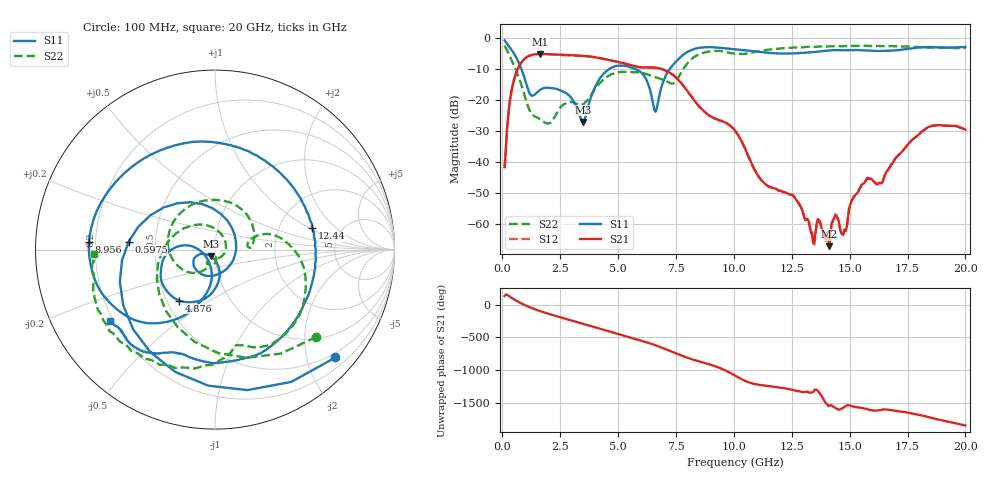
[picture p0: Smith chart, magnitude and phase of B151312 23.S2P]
!  2-Port S-parameters saved by WinCal
! VAR MeasName=S-Parameters (CALIBRATED_DATA) read from VNA (N5244A)
! VAR MeasDate=12/8/2015 5:45:11 PM
! VAR NAME=B151312 23
! VAR FILENAME=B151312 23.S2P
! VAR DATE=12/8/2015 5:45:11 PM
! VAR PHYS_PORTS=1,2
# Hz S DB R 50
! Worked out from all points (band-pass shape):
!   401 points, 100 MHz to 20 GHz, reference 50 ohm
!   highest |S21| = -5.26 dB at 1.642 GHz (marker M1); lowest = -67.2 dB at 14.13 GHz (marker M2)
!   |S21| within 3 dB of the highest: 802.2 MHz to 5.238 GHz (4.436 GHz wide, 147 % of centre)
!   lowest |S11| = -27.1 dB at 3.483 GHz (marker M3), VSWR 1.09, Z = 47.6 - j3.58 ohm
!   |S11| at or under -10 dB: 819.6 MHz to 4.642 GHz (3.823 GHz wide, 140 % of centre); 5.699 GHz to 7.241 GHz (1.542 GHz wide, 23.8 % of centre)
!   |S22| runs from -27.7 to -2.6 dB; largest |S21 - S12| = 0.0015
!   S11 on the Smith chart (normalised r, x): 100 MHz: 0.40, -2.56; 597.5 MHz: 0.35, +0.04; 4.876 GHz: 0.58, -0.37; 8.956 GHz: 0.17, +0.03; 12.44 GHz: 3.10, +1.06; 20 GHz: 0.19, -0.30
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1e8  -0.91 -41.9  -41.71 130.8  -42.02 132.5  -2.56 -40.8
3.4875e8  -3.41 -122.2  -19.30 114.8  -19.29 114.7  -6.40 -115.9
5.975e8  -6.31 175.0  -11.44 60.5  -11.44 60.5  -10.61 -178.0
1.04525e9  -15.12 66.6  -6.32 -19.8  -6.32 -19.8  -20.62 67.7
1.64225e9  -16.78 -93.1  -5.26 -101.4  -5.27 -101.4  -26.36 -77.8
2.43825e9  -16.78 -145.5  -5.50 172.5  -5.50 172.4  -23.16 -86.5
3.43325e9  -26.77 -134.7  -5.86 72.1  -5.86 72.1  -21.62 -121.7
3.483e9  -27.13 -121.5  -5.88 67.1  -5.88 67.1  -21.46 -119.5
4.12975e9  -14.18 -86.3  -6.47 0.2  -6.47 0.2  -15.37 -130.6
4.876e9  -9.20 -125.1  -7.62 -76.3  -7.62 -76.4  -11.36 165.3
5.82125e9  -10.37 -166.2  -9.38 -173.5  -9.36 -173.6  -11.19 76.1
6.7665e9  -19.17 -101.1  -9.88 77.8  -9.88 77.8  -13.10 12.7
7.91075e9  -4.98 -133.7  -16.36 -81.7  -16.34 -82.0  -9.07 12.4
8.9555e9  -3.06 176.3  -25.18 165.3  -25.17 164.8  -4.41 -41.3
1.005e10  -3.75 131.9  -29.91 -4.9  -29.96 -5.1  -5.15 -74.9
1.119425e10  -4.66 78.8  -45.94 -150.8  -45.92 -150.5  -4.23 -87.0
1.2438e10  -5.10 12.3  -50.55 145.5  -50.59 146.3  -3.29 -106.3
1.338325e10  -4.69 -32.1  -62.72 99.8  -63.71 98.5  -2.99 -117.7
1.41295e10  -4.13 -59.6  -67.17 -103.8  -66.77 -101.1  -2.83 -127.1
1.67165e10  -4.22 -111.1  -42.01 -169.4  -41.80 -168.8  -2.70 -153.0
1.835825e10  -3.06 -130.2  -28.96 85.7  -28.94 85.6  -3.19 -166.7
2e10  -3.01 -146.0  -29.62 -46.5  -29.68 -47.7  -3.39 -178.1
